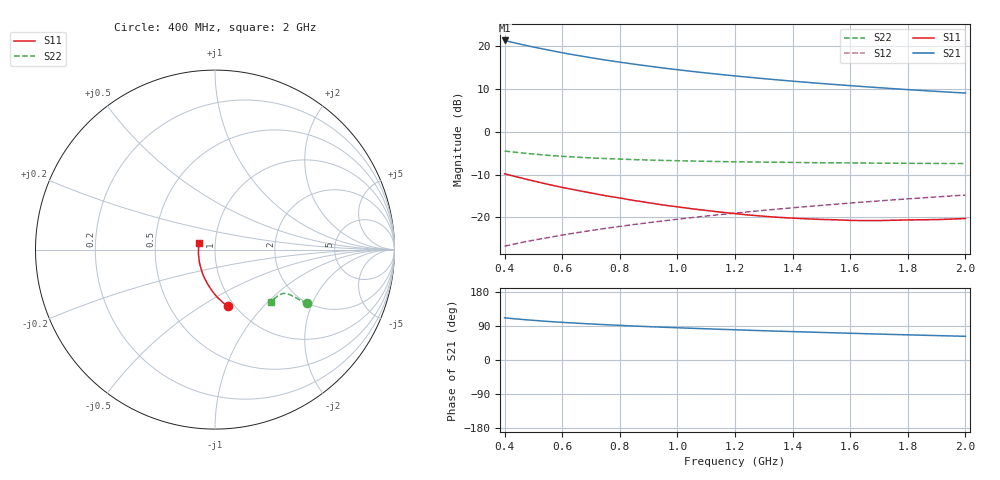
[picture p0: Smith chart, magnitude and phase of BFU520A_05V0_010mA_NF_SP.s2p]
! Filename:  P:\Prog\Test\Noise\ATS_data\Testdata_Net\06 Compressed Noise after Statistics\BFU520A_APG2013_30_A05_05p0V_010mA_NF_CM01_D.sf
! Date/Time: Wed 24/Apr/2013 20:06:18
! BFU520A_APG2013_30_A05_05p0V_1to20mA_NF_CM01_Bias6_R.sf
! Noise Parameter Data File
! BFU520A_APG2013_30_A05_05p0V_1to20mA_NF_CM01
! Date/time: Thu Apr 11 01:07:08 2013
! VAR V_out= 5.000000
! VAR I_out= 9.995000
! VAR V_in= 0.841700
! VAR I_in= 0.110905
! Device data file deembeded for feedlines and parallel
! Original file: \06 Compressed Noise after Statistics\BFU520A_APG2013_30_A05_05p0V_010mA_NF_CM01_R.sf
! Feed-files: PR017V01_150413_Feed1.s2p, PR017V01_150413_Feed2.s2p
! Parallel-file: PR017V01_150413_Par.s2p
# MHz S MA R 50
!  Freq-MHz  S11-mag  S11-arg  S21-mag  S21-arg  S12-mag  S12-arg  S22-mag  S22-arg
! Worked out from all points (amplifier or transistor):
!   37 points, 400 MHz to 2 GHz, reference 50 ohm
!   highest |S21| = 21.4 dB at 400 MHz (marker M1)
!   |S21| within 3 dB of that: start of sweep to 610.4 MHz
!   unconditionally stable (mu >= 1): 1.275 GHz to end of sweep
!   at 500 MHz: K = 0.82, MSG = 22.6 dB, |S12| = -25.4 dB
!   at 1.1 GHz: K = 0.99, MSG = 16.7 dB, |S12| = -19.7 dB
!   at 2 GHz: K = 1.00, MAG = 11.5 dB, |S12| = -14.8 dB
!   lowest NFmin = 0.83 dB at 420 MHz
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400  0.3225 -77.5  11.72 111.3  0.04586 68.6  0.596 -30.2
420  0.3099 -79.5  11.29 109.8  0.04749 68.6  0.5849 -30.4
440  0.2977 -81.6  10.89 108.4  0.04908 68.7  0.575 -30.4
460  0.2868 -83.3  10.5 107.1  0.05071 68.8  0.5659 -30.6
480  0.2763 -85.3  10.15 105.8  0.05226 68.9  0.5567 -30.6
500  0.2662 -87.1  9.815 104.7  0.05385 69.0  0.5492 -30.7
550  0.2428 -91.5  9.085 101.8  0.05777 69.3  0.5305 -30.7
600  0.2235 -95.5  8.418 99.4  0.06181 69.6  0.5168 -30.8
650  0.207 -99.2  7.856 97.2  0.06586 69.9  0.5049 -30.9
700  0.1923 -103.2  7.36 95.1  0.06992 70.2  0.4949 -30.9
750  0.1787 -106.9  6.918 93.2  0.07402 70.4  0.4863 -31.0
800  0.1679 -110.7  6.531 91.4  0.07814 70.6  0.4793 -31.2
850  0.157 -114.7  6.184 89.7  0.08229 70.7  0.4728 -31.4
950  0.1392 -122.3  5.585 86.5  0.09059 71.0  0.4627 -31.9
1050  0.1256 -129.8  5.095 83.7  0.09897 71.1  0.4545 -32.5
1150  0.1148 -138.4  4.687 81.0  0.1075 71.1  0.4483 -33.2
1200  0.1102 -142.2  4.508 79.8  0.1118 71.0  0.4459 -33.6
1350  0.09978 -154.7  4.045 76.0  0.1247 70.8  0.44 -35.0
1500  0.09423 -167.7  3.675 72.7  0.1377 70.4  0.4343 -36.6
1650  0.09137 -179.6  3.374 69.5  0.1509 69.8  0.4312 -38.4
1750  0.09218 172.5  3.197 67.4  0.1597 69.4  0.4287 -39.6
2000  0.09672 156.2  2.841 62.5  0.1819 68.2  0.4249 -43.1
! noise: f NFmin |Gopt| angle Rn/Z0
400  0.8666  0.0243  -168.9  0.1069
460  0.8559  0.04121  -170.9  0.0982
600  0.9643  0.02652  -117.1  0.1235
800  0.9162  0.07274  -170.8  0.0929
1000  0.9569  0.07327  -152  0.0923
1200  0.9671  0.09226  -150.3  0.0971
1400  0.9955  0.09833  -140.3  0.1016
1600  1.008  0.1311  -142.3  0.0957
1800  0.981  0.1587  -140.9  0.0931
2000  1  0.1861  -136.9  0.0935
